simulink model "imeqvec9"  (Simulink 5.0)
settings: Solver=ode45  StartTime=0.0  StopTime=1  MaxStep=5e-3  RelTol=1e-3
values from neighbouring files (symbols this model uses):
  H = 0.60    (= 0.6)    [IMabc2.m]    (also in IMcur0.m = 0.3; imdef0vec.m = 0.3; imdef1vec.m = 0.3; imdef2vec.m = 0.3)
  ic = [fs0 fr0]    [imdef0vec.m]    (also in imdef1vec.m; imdef2vec.m = F; imic2.m = [phids phiqs phidr phiqr n0]'; imic3.m = [phids phiqs phidr phiqr n0]')
  Lm = eval(get(hLm,'String'))    [im3d.m]    (also in IMabc2.m = 4.5; imabcparam.m = 0.0847; IMabcrun0.m = 0.0847; IMabcrun1.m = 0.0847)
  Lrl = eval(get(hLr,'String'))    [im3d.m]    (also in IMabc2.m = 0.1; imabcparam.m = 0.0025; IMabcrun0.m = 0.0025; IMabcrun1.m = 0.0025)
  Lsl = eval(get(hLs,'String'))    [im3d.m]    (also in IMabc2.m = 0.1; imabcparam.m = 0.0025; IMabcrun0.m = 0.0025; IMabcrun1.m = 0.0025)
  n0 = 0.98    [imdef0vec.m]    (also in imdef1vec.m = 0.978; imdef2vec.m; imdefrotflux.m; imdefSIvec1.m = 0.95)
  Rr = input('Rotor resistance)[default = 2] =')    [Actac.m]    (also in im1phase.m = 0.3; im3d.m = eval(get(hRr,'String')); IMabc2.m = 0.02; imabcparam.m = 0.408)
  Rs = eval(get(hRs,'String'))    [im3d.m]    (also in IMabc2.m = 0.01; imabcparam.m = 0.531; IMabcrun0.m = 0.531; IMabcrun1.m = 0.531)
  Tl0 = Is*conj(Is)*Req    [imdef0vec.m]    (also in imdef1vec.m; imdef2vec.m = Lm*(I(2)*I(3)-I(1)*I(4)); imdefrotflux.m; imdefSIvec1.m = Te0/To)
  vs = 1.0    (= 1)    [imdef0vec.m]    (also in imdef1vec.m; imdef2vec.m; imdefrotflux.m; imdefSIvec1.m)
  wk = ws    (= 1)    [imdef0vec.m]    (also in imdef1vec.m; imdef2vec.m; imdefrotflux.m; imdefSIvec1.m)
  wo = 2*pi*freq0    [calc0.m]    (also in IMabc2.m = 376.991118431; imabcparam.m = 376.991118431; IMabcrun0.m = 376.991118431; IMabcrun1.m = 376.991118431)

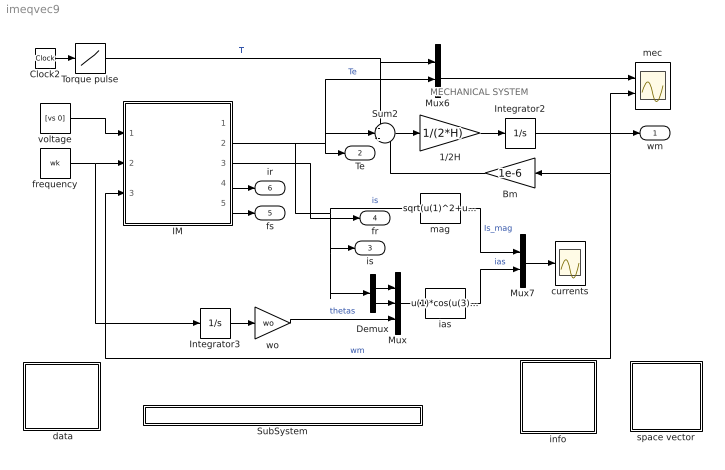
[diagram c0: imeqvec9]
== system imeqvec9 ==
  note: MECHANICAL SYSTEM
  " data" : Subsystem
  1/2H : Gain  Gain=1/(2*H)
  Bm : Gain  Orientation=left  Gain=1e-6
  Clock2 : Clock
  Demux : Demux  Outputs=2
  IM : Subsystem
  Integrator2 : Integrator  InitialCondition=n0
  Integrator3 : Integrator
  Mux : Mux  Inputs=3
  Mux6 : Mux  Inputs=2
  Mux7 : Mux  Inputs=2
  SubSystem : Subsystem
  Sum2 : Sum  Inputs=-+-
  Torque pulse : Lookup  InputValues=[0 0.2 0.2 0.6 0.6 2]  OutputValues="[Tl0 Tl0  .5 .5 1 1]"
  currents : Scope
  frequency : Constant  Value=wk
  ias : Fcn  Expr=u(1)*cos(u(3))-u(2)*sin(u(3))
  info : Subsystem
  mag : Fcn  Expr=sqrt(u(1)^2+u(2)^2)
  mec : Scope  NumInputPorts=2
  space vector : Subsystem
  voltage : Constant  Value=[vs 0]
  wo : Gain  Gain=wo
  wm : Outport
  Te : Outport  Port=2
  is : Outport  Port=3
  fr : Outport  Port=4
  fs : Outport  Port=5
  ir : Outport  Port=6
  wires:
  voltage/1 -> IM/1(vs)
  frequency/1 -> Integrator3/1, IM/2(wk)
  Demux/1 -> Mux/1
  Demux/2 -> Mux/2
  Mux/1 -> ias/1
  ias/1 -> Mux7/2  "ias"
  mag/1 -> Mux7/1  "Is_mag"
  Mux7/1 -> currents/1
  IM/2(is) -> mag/1, Demux/1, is/1  "is"
  Sum2/1 -> 1/2H/1
  1/2H/1 -> Integrator2/1
  Mux6/1 -> mec/1
  IM/1(Te) -> Sum2/2, Mux6/2, Te/1  "Te"
  Bm/1 -> Sum2/3
  Integrator3/1 -> wo/1
  wo/1 -> Mux/3  "thetas"
  Integrator2/1 -> mec/2, wm/1, IM/3(wm), Bm/1  "wm"
  Clock2/1 -> Torque pulse/1
  Torque pulse/1 -> Mux6/1, Sum2/1  "Tl"
  IM/3(fr) -> fr/1
  IM/5(fs) -> fs/1
  IM/4(ir) -> ir/1

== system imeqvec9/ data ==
  note: This demo simulates the running of an induction motor in steady-state when a sudden input change is effected: a)torque step changes at constant voltage excitation b) voltage input sag at constant frequency and load torque c)simultaneous step changes in voltage magnitude and frequency
  note: Double click the block to enter the machine parameters and initial conditions and then run the simulation

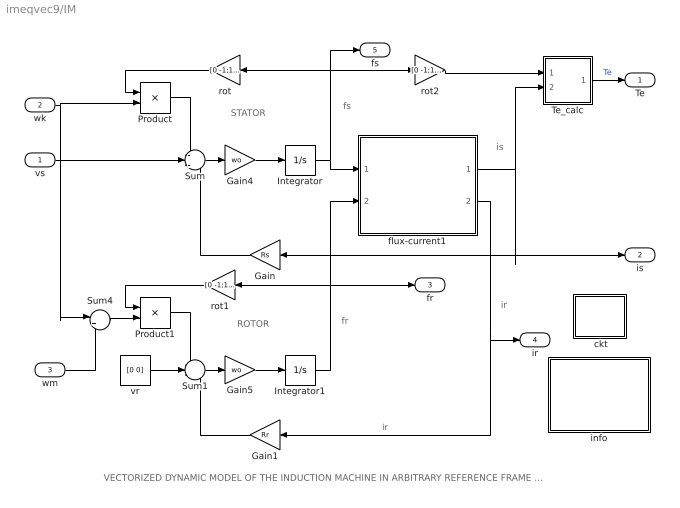
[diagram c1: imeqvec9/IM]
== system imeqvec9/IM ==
  note: ROTOR
  note: STATOR
  note: fs
  note: fr
  note: is
  note: VECTORIZED DYNAMIC MODEL OF THE INDUCTION MACHINE IN ARBITRARY REFERENCE FRAME (per unit formulation)
  note: ir
  vs : Inport
  wk : Inport  Port=2
  wm : Inport  Port=3
  " ckt" : Subsystem
  Gain : Gain  Orientation=left  Gain=Rs
  Gain1 : Gain  Orientation=left  Gain=Rr
  Gain4 : Gain  Gain=wo
  Gain5 : Gain  Gain=wo
  Integrator : Integrator  InitialCondition=[ic(1) ic(2)]
  Integrator1 : Integrator  InitialCondition=[ic(3) ic(4)]
  Product : Product
  Product1 : Product
  Sum : Sum  Inputs=-+-
  Sum1 : Sum  Inputs=-+-
  Sum4 : Sum  Inputs=|+-
  Te_calc : Subsystem
  flux-current1 : Subsystem
  info : Subsystem
  rot : Gain  Orientation=left  Gain=[0 -1;1 0]  Multiplication=Matrix(K*u)
  rot1 : Gain  Orientation=left  Gain=[0 -1;1 0]  Multiplication=Matrix(K*u)
  rot2 : Gain  Gain=[0 -1;1 0]  Multiplication=Matrix(K*u)
  vr : Constant  Value=[0 0]
  Te : Outport
  is : Outport  Port=2
  fr : Outport  Port=3
  ir : Outport  Port=4
  fs : Outport  Port=5
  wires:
  Gain/1 -> Sum/3
  vr/1 -> Sum1/2
  Gain1/1 -> Sum1/3
  flux-current1/2(ir) -> Gain1/1, ir/1  "ir"
  Integrator/1 -> flux-current1/1(fs), rot/1, rot2/1, fs/1
  Integrator1/1 -> rot1/1, flux-current1/2(fr), fr/1
  Product1/1 -> Sum1/1
  rot1/1 -> Product1/1
  Product/1 -> Sum/1
  rot/1 -> Product/1
  rot2/1 -> Te_calc/1(fs)
  Sum4/1 -> Product1/2
  Sum/1 -> Gain4/1
  Gain4/1 -> Integrator/1
  Sum1/1 -> Gain5/1
  Gain5/1 -> Integrator1/1
  flux-current1/1(is) -> Te_calc/2(is), Gain/1, is/1
  Te_calc/1(Te) -> Te/1  "Te"
  vs/1 -> Sum/2
  wk/1 -> Product/2, Sum4/1
  wm/1 -> Sum4/2

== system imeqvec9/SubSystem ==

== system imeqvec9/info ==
  note: The induction machine is modeled in vectorized form in conformity with the state vector formulation. This one-to-one correspondence can be seen by clicking both the INDUCTION MACHINE subsystem block and the MATHEMATICAL MODEL equation block. The synchronous reference frame is chosen here because the machine is operating under balanced three-phase sinusoidal excitation; the input voltage is thefore constant as indicated. The parameters describing the electromechanical system are expressed in per unit and are entered after double-clicking one of the PARAMETERS/IC blocks. The system is initially assumed to be operated under load in a steady state defined by a specified speed. The initial conditions are established by calling a phasor calculation based on the standard steady-state equivalent circuit of the induction machine. The simulation can then be run. In the present case, it exhibits the dynamic response to a pulsed applied torque. The torque developed, the speed, and the stator current are observed on the scopes . The torque-speed dynamic characteristics can then be obtained after double clicking the X-Y PLOT block.
  note: Running of a Line-Fed Induction Motor Synchronous frame Per unit system

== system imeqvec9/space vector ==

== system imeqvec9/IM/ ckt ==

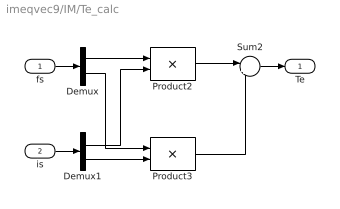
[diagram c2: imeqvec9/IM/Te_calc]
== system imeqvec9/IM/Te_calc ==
  fs : Inport
  is : Inport  Port=2
  Demux : Demux  Outputs=2
  Demux1 : Demux  Outputs=2
  Product2 : Product
  Product3 : Product
  Sum2 : Sum  Inputs=|++
  Te : Outport
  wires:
  Demux/1 -> Product2/1
  Demux1/2 -> Product3/2
  Demux/2 -> Product3/1
  Demux1/1 -> Product2/2
  Product2/1 -> Sum2/1
  Product3/1 -> Sum2/2
  Sum2/1 -> Te/1
  fs/1 -> Demux/1
  is/1 -> Demux1/1

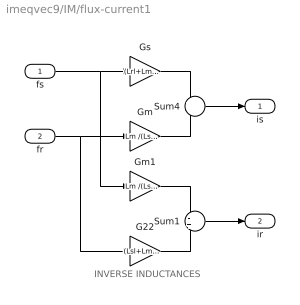
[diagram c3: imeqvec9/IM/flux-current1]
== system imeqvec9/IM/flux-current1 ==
  note: INVERSE INDUCTANCES
  fs : Inport
  fr : Inport  Port=2
  G22 : Gain  Gain=(Lsl+Lm )/(Lsl*Lrl+Lsl*Lm+Lrl*Lm)
  Gm : Gain  Gain=Lm /(Lsl*Lrl+Lsl*Lm+Lrl*Lm)
  Gm1 : Gain  Gain=Lm /(Lsl*Lrl+Lsl*Lm+Lrl*Lm)
  Gs : Gain  Gain=(Lrl+Lm) /(Lsl*Lrl+Lsl*Lm+Lrl*Lm)
  Sum1 : Sum  Inputs=-+
  Sum4 : Sum  Inputs=+-
  is : Outport
  ir : Outport  Port=2
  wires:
  fs/1 -> Gs/1, Gm1/1
  Gs/1 -> Sum4/1
  fr/1 -> Gm/1, G22/1
  Gm/1 -> Sum4/2
  Sum4/1 -> is/1
  Gm1/1 -> Sum1/1
  G22/1 -> Sum1/2
  Sum1/1 -> ir/1

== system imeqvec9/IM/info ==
  note: Mathematical model of the induction machine. Space vector formulation in an arbitrary dq common reference frame. Per unit description.
  note: Electrical system equations: vs = Rs is + 1/wo (dfs/dt) + wk M(pi/2) fs vr = Rr ir + 1/wo (dfr/dt) + (wk - wm) M(pi/2) fr where the variables i, v, and f are 2-dimensional space vectors; for instance is = [ids iqs] and so forth, wk is the speed of the reference frame, wm the rotor speed, and M(pi/2)represents a 90o space rotator namely M(pi/2) = [0 -1;1 0] The flux linkage current relations are: fs = Ls is + Lm ir fr = Lm is + Lr ir where Ls =Lm +Lsl and Lr = Lm +Lrl Mechanical system equations: Te = 2H (dwm/dt ) + Bm wm + Tl where Te = fs (cross) is = M(pi/2) fs (dot) is = fds iqs - fqs ids = fs x is = M(pi/2) fs . is = ir x fr = Lm (ir x is) = Lm/Lr (fr x is) = 1/Lm' (fr x fs) Lm' =Lm c/(1-c) c = 1 - Lm^2/(Ls Lr)
